FUNCTION "TAVOLA 1" : VOID
TITLE =TAVOLE DI SOLLEVAMENTO
AUTHOR : LD
FAMILY : DESTECK
NAME : TAVOLA
VERSION : 0.1

BEGIN
NETWORK
TITLE =Tavola 1: Antischiacciamento in corso
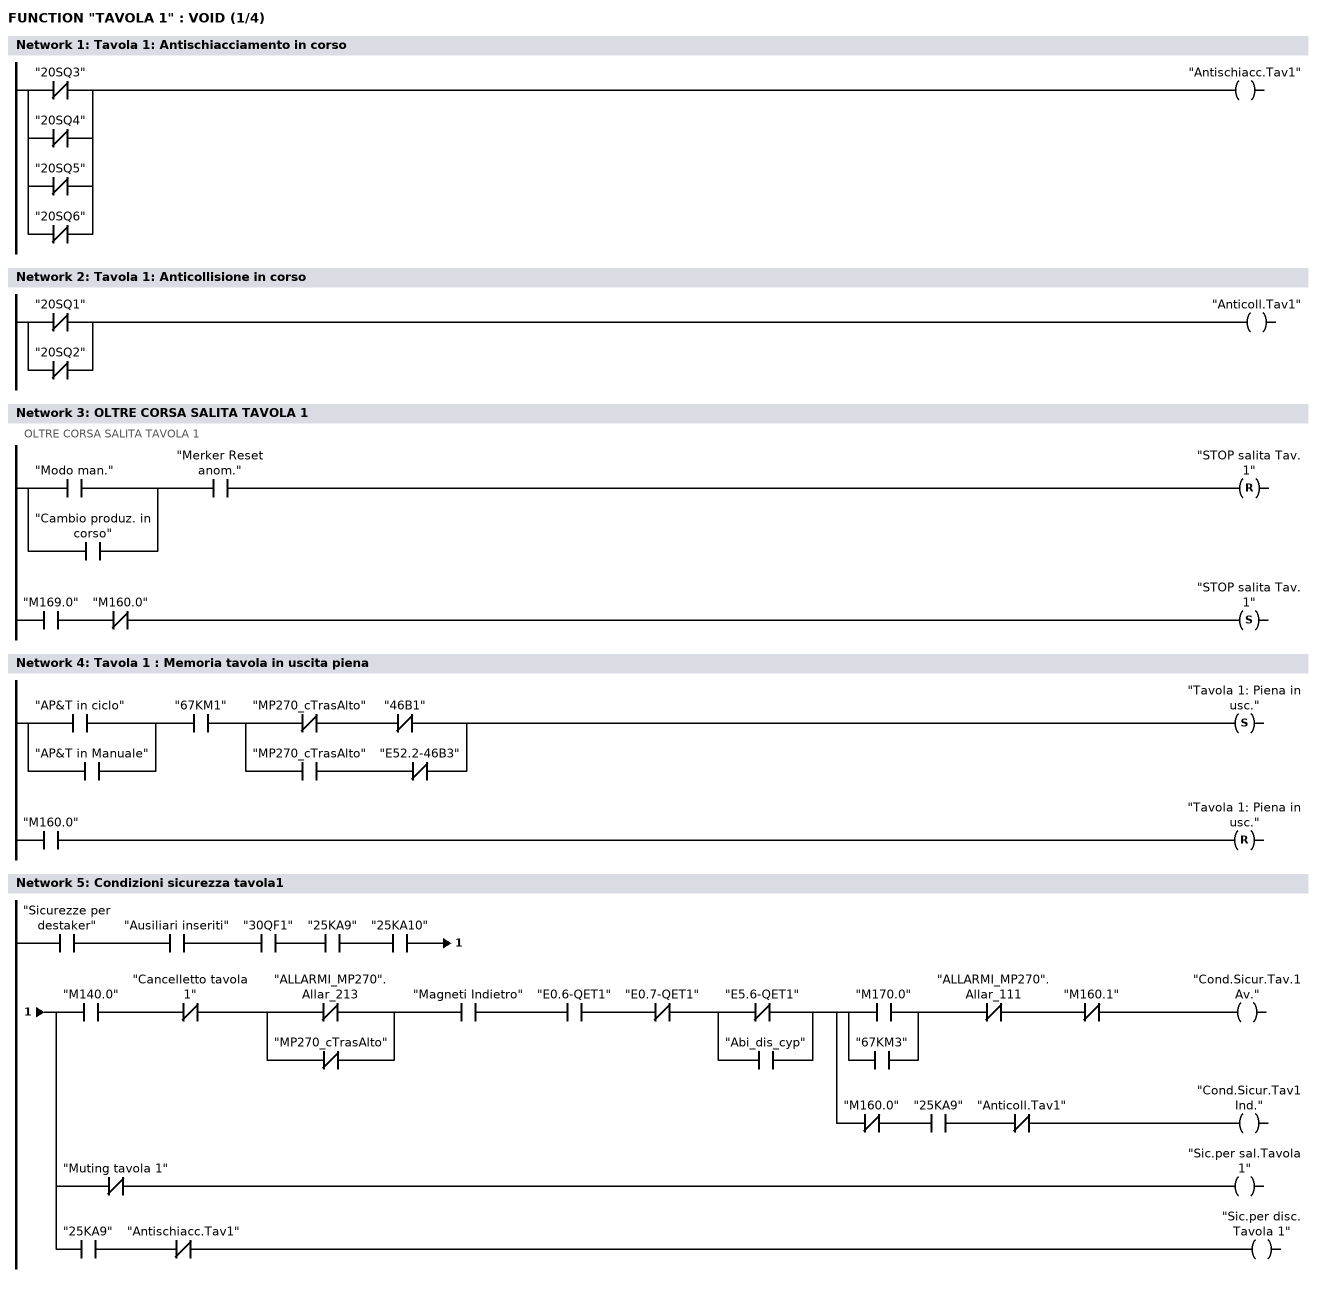
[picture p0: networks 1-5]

      ON    "20SQ3";
      ON    "20SQ4";
      ON    "20SQ5";
      ON    "20SQ6";
      =     "Antischiacc.Tav1";
NETWORK
TITLE =Tavola 1: Anticollisione in corso

      ON    "20SQ1";
      ON    "20SQ2";
      =     "Anticoll.Tav1";
NETWORK
TITLE =OLTRE CORSA SALITA TAVOLA 1
//OLTRE CORSA SALITA TAVOLA 1
      U(    ;
      O     "Modo man.";
      O     "Cambio produz. in corso";
      )     ;
      U     "Merker Reset anom.";
      R     "STOP salita Tav. 1";
      U     "M169.0";
      UN    "M160.0";
      S     "STOP salita Tav. 1";
      NOP   0;
NETWORK
TITLE =Tavola 1 : Memoria tavola in uscita piena

      U(    ;
      O     "AP&T  in ciclo";
      O     "AP&T in Manuale";
      )     ;
      U     "67KM1";
      U(    ;
      UN    "MP270_cTrasAlto";
      UN    "46B1";
      O     ;
      U     "MP270_cTrasAlto";
      UN    "E52.2-46B3";
      )     ;
      S     "Tavola 1: Piena in usc.";
      U     "M160.0";
      R     "Tavola 1: Piena in usc.";
      NOP   0;
NETWORK
TITLE =Condizioni sicurezza tavola1

      U     "Sicurezze per destaker";
      U     "Ausiliari inseriti";
      U     "30QF1";
      U     "25KA9";
      U     "25KA10";
      =     L      0.0;
      U     L      0.0;
      U     "M140.0";
      UN    "Cancelletto tavola 1";
      U(    ;
      ON    "ALLARMI_MP270".Allar_213;
      ON    "MP270_cTrasAlto";
      )     ;
      U     "Magneti Indietro";
      U     "E0.6-QET1";
      UN    "E0.7-QET1";
      U(    ;
      ON    "E5.6-QET1";
      O     "Abi_dis_cyp";
      )     ;
      =     L      0.1;
      U     L      0.1;
      U(    ;
      O     "M170.0";
      O     "67KM3";
      )     ;
      UN    "ALLARMI_MP270".Allar_111;
      UN    "M160.1";
      =     "Cond.Sicur.Tav.1 Av.";
      U     L      0.1;
      UN    "M160.0";
      U     "25KA9";
      UN    "Anticoll.Tav1";
      =     "Cond.Sicur.Tav1 Ind.";
      U     L      0.0;
      UN    "Muting tavola 1";
      =     "Sic.per sal.Tavola 1";
      U     L      0.0;
      U     "25KA9";
      UN    "Antischiacc.Tav1";
      =     "Sic.per disc. Tavola 1";
NETWORK
TITLE =MEMORIA QUOTA RAGGIUNTA TAVOLA
//MEMORIA QUOTA RAGGIUNTA TAVOLA
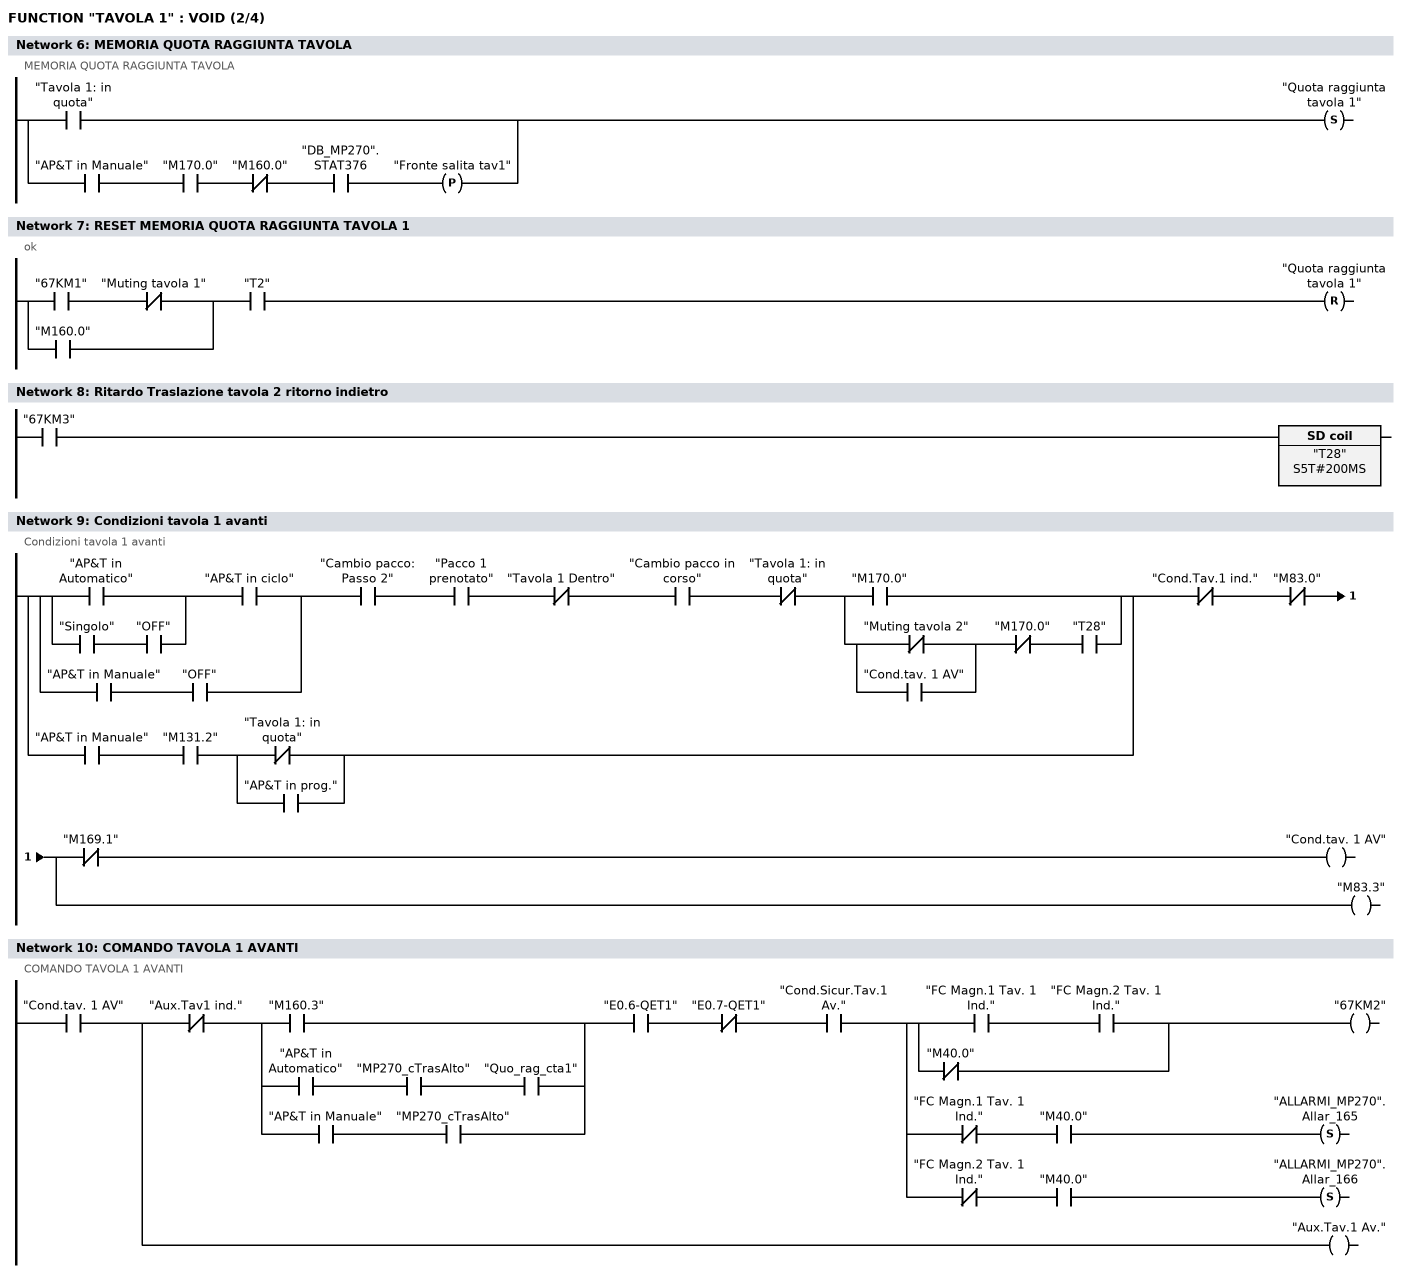
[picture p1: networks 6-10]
      O     "Tavola 1: in quota";
      O(    ;
      U     "AP&T in Manuale";
      U     "M170.0";
      UN    "M160.0";
      U     "DB_MP270".STAT376;
      FP    "Fronte salita tav1";
      )     ;
      S     "Quota raggiunta tavola 1";
NETWORK
TITLE =RESET MEMORIA QUOTA RAGGIUNTA TAVOLA 1
//ok
      U(    ;
      U     "67KM1";
      UN    "Muting tavola 1";
      O     "M160.0";
      )     ;
      U     "T2";
      R     "Quota raggiunta tavola 1";
NETWORK
TITLE =Ritardo Traslazione tavola 2 ritorno indietro

      U     "67KM3";
      L     S5T#200MS;
      SE    "T28";
NETWORK
TITLE =Condizioni tavola 1 avanti
//Condizioni tavola 1 avanti
      U(    ;
      U(    ;
      U(    ;
      O     "AP&T in Automatico";
      O     ;
      U     "Singolo";
      U     "OFF";
      )     ;
      U     "AP&T  in ciclo";
      O     ;
      U     "AP&T in Manuale";
      U     "OFF";
      )     ;
      U     "Cambio pacco: Passo 2";
      U     "Pacco 1 prenotato";
      UN    "Tavola 1 Dentro";
      U     "Cambio pacco in corso";
      UN    "Tavola 1: in quota";
      U(    ;
      O     "M170.0";
      O     ;
      U(    ;
      ON    "Muting tavola 2";
      O     "Cond.tav. 1 AV";
      )     ;
      UN    "M170.0";
      U     "T28";
      )     ;
      O     ;
      U     "AP&T in Manuale";
      U     "M131.2";
      U(    ;
      ON    "Tavola 1: in quota";
      O     "AP&T in prog.";
      )     ;
      )     ;
      UN    "Cond.Tav.1 ind.";
      UN    "M83.0";
      =     L      0.0;
      U     L      0.0;
      UN    "M169.1";
      =     "Cond.tav. 1 AV";
      U     L      0.0;
      BLD   102;
      =     "M83.3";
NETWORK
TITLE = COMANDO TAVOLA 1 AVANTI
// COMANDO TAVOLA 1 AVANTI
      U     "Cond.tav. 1 AV";
      =     L      0.0;
      U     L      0.0;
      UN    "Aux.Tav1 ind.";
      U(    ;
      O     "M160.3";
      O     ;
      U     "AP&T in Automatico";
      U     "MP270_cTrasAlto";
      U     "Quo_rag_cta1";
      O     ;
      U     "AP&T in Manuale";
      U     "MP270_cTrasAlto";
      )     ;
      U     "E0.6-QET1";
      UN    "E0.7-QET1";
      U     "Cond.Sicur.Tav.1 Av.";
      =     L      0.1;
      U     L      0.1;
      U(    ;
      U     "FC Magn.1 Tav. 1 Ind.";
      U     "FC Magn.2 Tav. 1 Ind.";
      ON    "M40.0";
      )     ;
      =     "67KM2";
      U     L      0.1;
      UN    "FC Magn.1 Tav. 1 Ind.";
      U     "M40.0";
      S     "ALLARMI_MP270".Allar_165;
      U     L      0.1;
      UN    "FC Magn.2 Tav. 1 Ind.";
      U     "M40.0";
      S     "ALLARMI_MP270".Allar_166;
      U     L      0.0;
      BLD   102;
      =     "Aux.Tav.1 Av.";
NETWORK
TITLE =Condizioni tavola 1 indietro
//Condizioni tavola 1 indietro
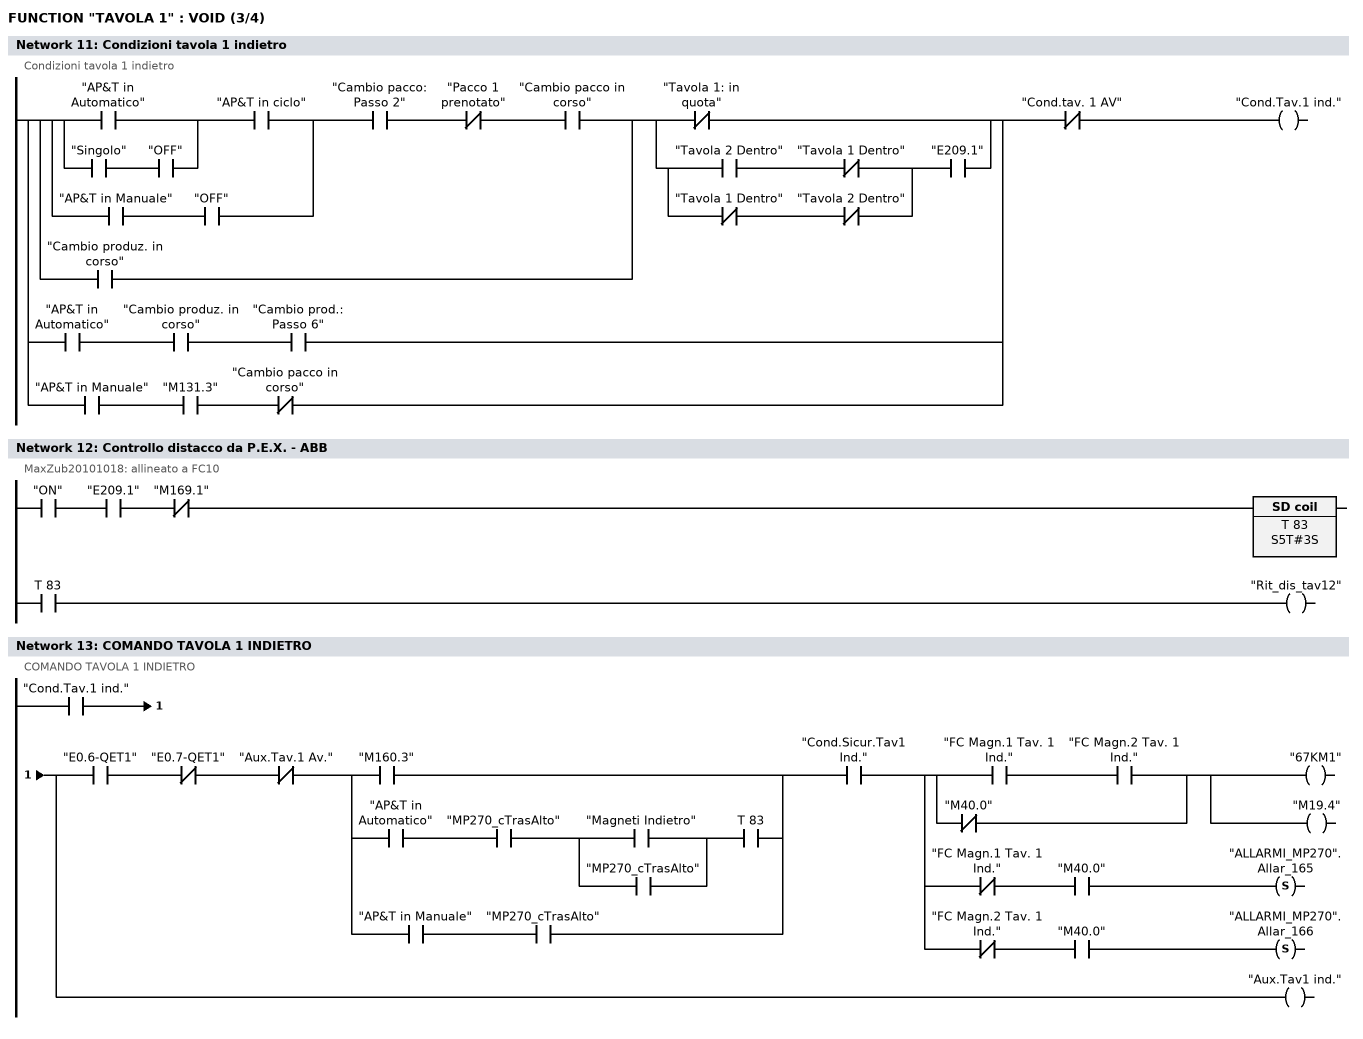
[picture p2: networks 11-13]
      U(    ;
      U(    ;
      U(    ;
      U(    ;
      O     "AP&T in Automatico";
      O     ;
      U     "Singolo";
      U     "OFF";
      )     ;
      U     "AP&T  in ciclo";
      O     ;
      U     "AP&T in Manuale";
      U     "OFF";
      )     ;
      U     "Cambio pacco: Passo 2";
      UN    "Pacco 1 prenotato";
      U     "Cambio pacco in corso";
      O     "Cambio produz. in corso";
      )     ;
      U(    ;
      ON    "Tavola 1: in quota";
      O     ;
      U(    ;
      U     "Tavola 2 Dentro";
      UN    "Tavola 1 Dentro";
      O     ;
      UN    "Tavola 1 Dentro";
      UN    "Tavola 2 Dentro";
      )     ;
      U     "E209.1";
      )     ;
      O     ;
      U     "AP&T in Automatico";
      U     "Cambio produz. in corso";
      U     "Cambio prod.: Passo 6";
      O     ;
      U     "AP&T in Manuale";
      U     "M131.3";
      UN    "Cambio pacco in corso";
      )     ;
      UN    "Cond.tav. 1 AV";
      =     "Cond.Tav.1 ind.";
NETWORK
TITLE =Controllo distacco da P.E.X. - ABB
//MaxZub20101018: allineato a FC10
      U     "ON";
      U     "E209.1";
      UN    "M169.1";
      L     S5T#3S;
      SE    T     83;
      NOP   0;
      NOP   0;
      NOP   0;
      U     T     83;
      =     "Rit_dis_tav12";
NETWORK
TITLE =COMANDO TAVOLA 1 INDIETRO
//COMANDO TAVOLA 1 INDIETRO
      U     "Cond.Tav.1 ind.";
      =     L      0.0;
      U     L      0.0;
      U     "E0.6-QET1";
      UN    "E0.7-QET1";
      UN    "Aux.Tav.1 Av.";
      U(    ;
      O     "M160.3";
      O     ;
      U     "AP&T in Automatico";
      U     "MP270_cTrasAlto";
      U(    ;
      O     "Magneti Indietro";
      O     "MP270_cTrasAlto";
      )     ;
      U     T     83;
      O     ;
      U     "AP&T in Manuale";
      U     "MP270_cTrasAlto";
      )     ;
      U     "Cond.Sicur.Tav1 Ind.";
      =     L      0.1;
      U     L      0.1;
      U(    ;
      U     "FC Magn.1 Tav. 1 Ind.";
      U     "FC Magn.2 Tav. 1 Ind.";
      ON    "M40.0";
      )     ;
      =     "67KM1";
      =     "M19.4";
      U     L      0.1;
      UN    "FC Magn.1 Tav. 1 Ind.";
      U     "M40.0";
      S     "ALLARMI_MP270".Allar_165;
      U     L      0.1;
      UN    "FC Magn.2 Tav. 1 Ind.";
      U     "M40.0";
      S     "ALLARMI_MP270".Allar_166;
      U     L      0.0;
      BLD   102;
      =     "Aux.Tav1 ind.";
NETWORK
TITLE =Condizioni salita tavola 1
//Condizioni salita tavola 1
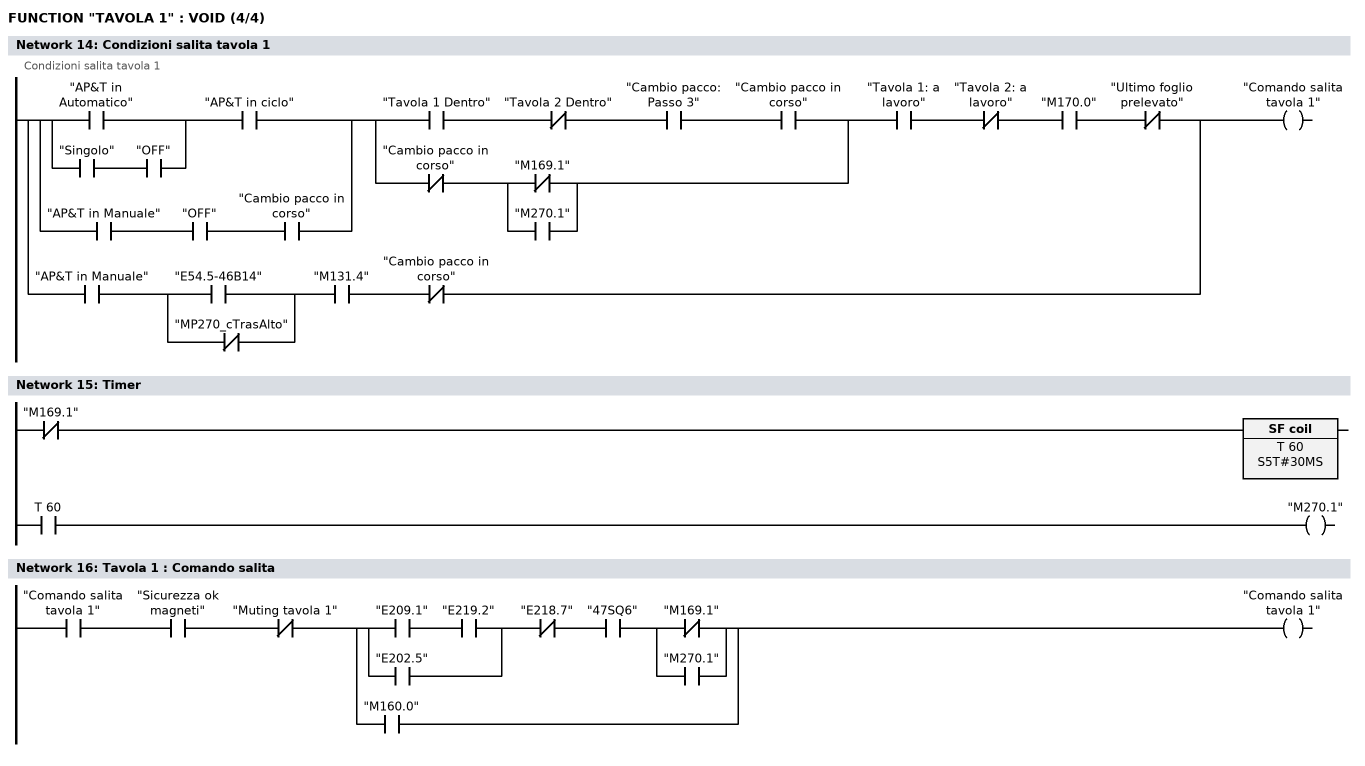
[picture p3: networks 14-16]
      U(    ;
      U(    ;
      O     "AP&T in Automatico";
      O     ;
      U     "Singolo";
      U     "OFF";
      )     ;
      U     "AP&T  in ciclo";
      O     ;
      U     "AP&T in Manuale";
      U     "OFF";
      U     "Cambio pacco in corso";
      )     ;
      U(    ;
      U     "Tavola 1 Dentro";
      UN    "Tavola 2 Dentro";
      U     "Cambio pacco: Passo 3";
      U     "Cambio pacco in corso";
      O     ;
      UN    "Cambio pacco in corso";
      U(    ;
      ON    "M169.1";
      O     "M270.1";
      )     ;
      )     ;
      U     "Tavola 1: a  lavoro";
      UN    "Tavola 2: a  lavoro";
      U     "M170.0";
      UN    "Ultimo foglio prelevato";
      O     ;
      U     "AP&T in Manuale";
      U(    ;
      O     "E54.5-46B14";
      ON    "MP270_cTrasAlto";
      )     ;
      U     "M131.4";
      UN    "Cambio pacco in corso";
      =     "Comando salita tavola 1";
NETWORK
TITLE =Timer

      UN    "M169.1";
      L     S5T#30MS;
      SA    T     60;
      NOP   0;
      NOP   0;
      NOP   0;
      U     T     60;
      =     "M270.1";
NETWORK
TITLE =Tavola 1 : Comando salita

      U     "Comando salita tavola 1";
      U     "Sicurezza ok magneti";
      UN    "Muting tavola 1";
      U(    ;
      U(    ;
      U     "E209.1";
      U     "E219.2";
      O     "E202.5";
      )     ;
      UN    "E218.7";
      U     "47SQ6";
      U(    ;
      ON    "M169.1";
      O     "M270.1";
      )     ;
      O     "M160.0";
      )     ;
      =     "Comando salita tavola 1";
NETWORK
TITLE =COMANDO SALITA TAVOLA 1
//COMANDO SALITA TAVOLA 1
//MaxZub20101018: ins. condizione per sollevamanto ritardato in cambio pacchi
      U(    ;
      U     "Comando salita tavola 1";
      UN    "Cambio pacco in corso";
      O(    ;
      U     "Comando salita tavola 1";
      U     "Cambio pacco in corso";
      L     S5T#2S;
      SE    "T43";
      NOP   0;
      NOP   0;
      NOP   0;
      U     "T43";
      )     ;
      O     ;
      U     "AP&T in Automatico";
      U     "MP270_cTrasAlto";
      U     "M160.0";
      U     "Mem_sal_pan1";
      )     ;
      U     "Sic.per sal.Tavola 1";
      UN    "STOP salita Tav. 1";
      U     "47SQ3";
      =     "78YV1A";
NETWORK
TITLE =Condizioni discesa tavola 1
//Condizioni discesa tavola 1
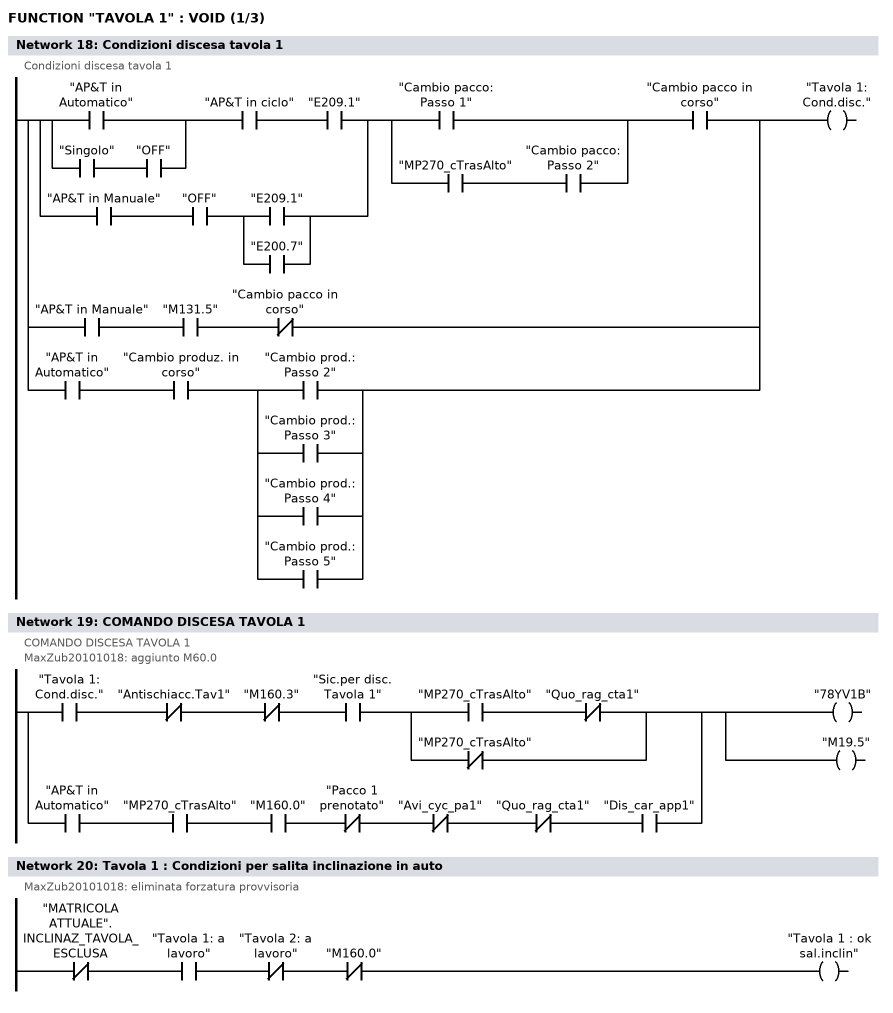
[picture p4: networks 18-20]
      U(    ;
      U(    ;
      O     "AP&T in Automatico";
      O     ;
      U     "Singolo";
      U     "OFF";
      )     ;
      U     "AP&T  in ciclo";
      U     "E209.1";
      O     ;
      U     "AP&T in Manuale";
      U     "OFF";
      U(    ;
      O     "E209.1";
      O     "E200.7";
      )     ;
      )     ;
      U(    ;
      O     "Cambio pacco: Passo 1";
      O     ;
      U     "MP270_cTrasAlto";
      U     "Cambio pacco: Passo 2";
      )     ;
      U     "Cambio pacco in corso";
      O     ;
      U     "AP&T in Manuale";
      U     "M131.5";
      UN    "Cambio pacco in corso";
      O     ;
      U     "AP&T in Automatico";
      U     "Cambio produz. in corso";
      U(    ;
      O     "Cambio prod.: Passo 2";
      O     "Cambio prod.: Passo 3";
      O     "Cambio prod.: Passo 4";
      O     "Cambio prod.: Passo 5";
      )     ;
      =     "Tavola 1: Cond.disc.";
NETWORK
TITLE =COMANDO DISCESA TAVOLA 1
//COMANDO DISCESA TAVOLA 1
//MaxZub20101018: aggiunto M60.0
      U     "Tavola 1: Cond.disc.";
      UN    "Antischiacc.Tav1";
      UN    "M160.3";
      U     "Sic.per disc. Tavola 1";
      U(    ;
      U     "MP270_cTrasAlto";
      UN    "Quo_rag_cta1";
      ON    "MP270_cTrasAlto";
      )     ;
      O     ;
      U     "AP&T in Automatico";
      U     "MP270_cTrasAlto";
      U     "M160.0";
      UN    "Pacco 1 prenotato";
      UN    "Avi_cyc_pa1";
      UN    "Quo_rag_cta1";
      U     "Dis_car_app1";
      =     "78YV1B";
      =     "M19.5";
NETWORK
TITLE =Tavola 1 : Condizioni per salita inclinazione in auto
//MaxZub20101018: eliminata forzatura provvisoria
      UN    "MATRICOLA ATTUALE".INCLINAZ_TAVOLA_ESCLUSA;
      U     "Tavola 1: a  lavoro";
      UN    "Tavola 2: a  lavoro";
      UN    "M160.0";
      =     "Tavola 1 : ok sal.inclin";
NETWORK
TITLE =Inclinazione tavola 1 sollevamento su
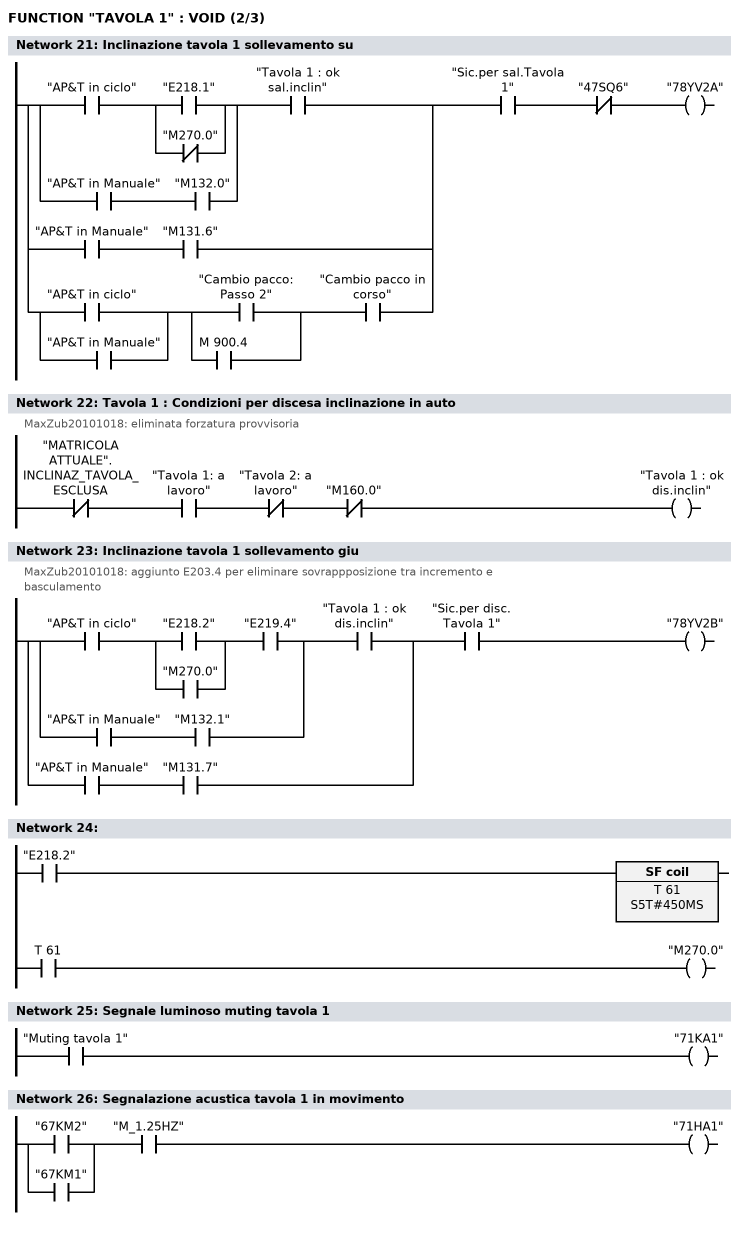
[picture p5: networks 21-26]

      U(    ;
      U(    ;
      U     "AP&T  in ciclo";
      U(    ;
      O     "E218.1";
      ON    "M270.0";
      )     ;
      O     ;
      U     "AP&T in Manuale";
      U     "M132.0";
      )     ;
      U     "Tavola 1 : ok sal.inclin";
      O     ;
      U     "AP&T in Manuale";
      U     "M131.6";
      O     ;
      U(    ;
      O     "AP&T  in ciclo";
      O     "AP&T in Manuale";
      )     ;
      U(    ;
      O     "Cambio pacco: Passo 2";
      O     M    900.4;
      )     ;
      U     "Cambio pacco in corso";
      )     ;
      U     "Sic.per sal.Tavola 1";
      UN    "47SQ6";
      =     "78YV2A";
NETWORK
TITLE =Tavola 1 : Condizioni per discesa inclinazione in auto
//MaxZub20101018: eliminata forzatura provvisoria
      UN    "MATRICOLA ATTUALE".INCLINAZ_TAVOLA_ESCLUSA;
      U     "Tavola 1: a  lavoro";
      UN    "Tavola 2: a  lavoro";
      UN    "M160.0";
      =     "Tavola 1 : ok dis.inclin";
NETWORK
TITLE =Inclinazione tavola 1 sollevamento giu
//MaxZub20101018: aggiunto E203.4 per eliminare sovrappposizione tra incremento e
//basculamento
      U(    ;
      U(    ;
      U     "AP&T  in ciclo";
      U(    ;
      O     "E218.2";
      O     "M270.0";
      )     ;
      U     "E219.4";
      O     ;
      U     "AP&T in Manuale";
      U     "M132.1";
      )     ;
      U     "Tavola 1 : ok dis.inclin";
      O     ;
      U     "AP&T in Manuale";
      U     "M131.7";
      )     ;
      U     "Sic.per disc. Tavola 1";
      =     "78YV2B";
NETWORK
TITLE =

      U     "E218.2";
      L     S5T#450MS;
      SA    T     61;
      NOP   0;
      NOP   0;
      NOP   0;
      U     T     61;
      =     "M270.0";
NETWORK
TITLE =Segnale luminoso muting tavola 1

      U     "Muting tavola 1";
      =     "71KA1";
NETWORK
TITLE =Segnalazione acustica tavola 1 in movimento

      U(    ;
      O     "67KM2";
      O     "67KM1";
      )     ;
      U     "M_1.25HZ";
      =     "71HA1";
NETWORK
TITLE =COMANDO POMPA TAVOLA 1
//COMANDO POMPA TAVOLA 1
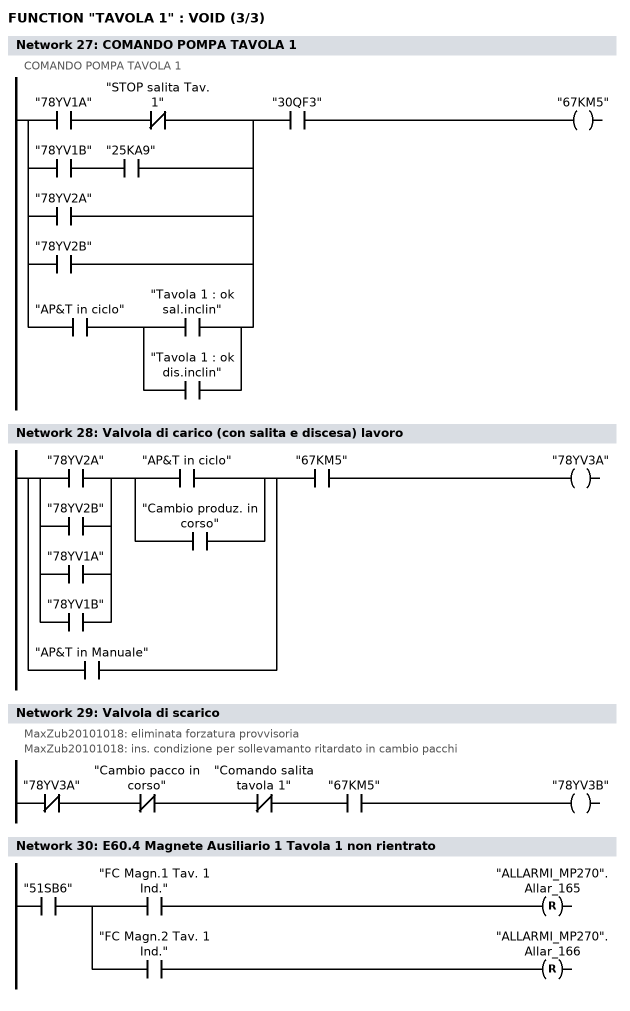
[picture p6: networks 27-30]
      U(    ;
      U     "78YV1A";
      UN    "STOP salita Tav. 1";
      O     ;
      U     "78YV1B";
      U     "25KA9";
      O     "78YV2A";
      O     "78YV2B";
      O     ;
      U     "AP&T  in ciclo";
      U(    ;
      O     "Tavola 1 : ok sal.inclin";
      O     "Tavola 1 : ok dis.inclin";
      )     ;
      )     ;
      U     "30QF3";
      =     "67KM5";
NETWORK
TITLE =Valvola di carico (con salita e discesa) lavoro

      U(    ;
      U(    ;
      O     "78YV2A";
      O     "78YV2B";
      O     "78YV1A";
      O     "78YV1B";
      )     ;
      U(    ;
      O     "AP&T  in ciclo";
      O     "Cambio produz. in corso";
      )     ;
      O     "AP&T in Manuale";
      )     ;
      U     "67KM5";
      =     "78YV3A";
NETWORK
TITLE =Valvola di scarico
//MaxZub20101018: eliminata forzatura provvisoria
//MaxZub20101018: ins. condizione per sollevamanto ritardato in cambio pacchi
//
      UN    "78YV3A";
      UN    "Cambio pacco in corso";
      UN    "Comando salita tavola 1";
      U     "67KM5";
      =     "78YV3B";
NETWORK
TITLE =E60.4 Magnete Ausiliario 1 Tavola 1 non rientrato

      U     "51SB6";
      =     L      0.0;
      U     L      0.0;
      U     "FC Magn.1 Tav. 1 Ind.";
      R     "ALLARMI_MP270".Allar_165;
      U     L      0.0;
      U     "FC Magn.2 Tav. 1 Ind.";
      R     "ALLARMI_MP270".Allar_166;
END_FUNCTION

